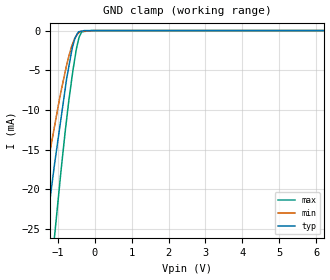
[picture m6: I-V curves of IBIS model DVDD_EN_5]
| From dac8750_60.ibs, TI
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[Model] DVDD_EN_5  |5V digital input
Model_type   Input
Vinl = 0.8
Vinh = 2
|   typ   min   max
|   (nom PVT)   (Fast PVT)   (slow PVT)
C_comp   1.528E-12   1.528E-12   1.528E-12
| Where   nom PVT is  Nominal Process, 5.0V, 36C
|   Fast PVT is Strong Process, 5.5V, -40C
|   Slow PVT is Weak Process, 4.5V, 134C
|C_comp - from L-C Tank method, L = 1nH, peak frequency
[Voltage Range]   5   4.5   5.5
|Operating Temperature   27   125   -40
|Junction Temperature
[Temperature Range]   36   134   -40
[Power Clamp Reference]   5   4.5   5.5
[GND Clamp Reference]   0   0   0
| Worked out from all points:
|   GND clamp passes 1 mA (typ) near -0.53 V on its own axis
[GND Clamp]
|   Voltage   I(typ)   I(min)   I(max)
-5V       -672.9mA   -540.5mA   -785.8mA
-1.516V   -35.58mA   -24.81mA   -50.62mA
-1.451V   -31.4mA    -22.74mA   -44.79mA
-1.252V   -22.88mA   -16.39mA   -33.85mA
-1.079V   -16.64mA   -11.93mA   -25.67mA
-796.6mV  -7.362mA   -5.208mA   -12.72mA
-605.8mV  -2.213mA   -1.79mA    -5.658mA
-530.3mV  -946.6uA   -922.1uA   -3.368mA
-427.8mV  -146.3uA   -282.7uA   -988.4uA
-349.4mV  -67.4uA    -95.14uA   -154.6uA
-106.1mV  -731.9nA   -29.92uA   0A
9.985V    0A         0A         0A
[POWER Clamp]
|   SCR cell for ESD function. Effects occurr above VDD x 2
|   Voltage   I(typ)   I(min)   I(max)
-5V       0A         0A         0A
0V        0A         0A         0A
10V       0A         0A         0A
